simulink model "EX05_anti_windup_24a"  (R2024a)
settings: Solver=VariableStepAuto  StartTime=0.0  StopTime=0.1  MaxStep=1e-5  RelTol=1e-5

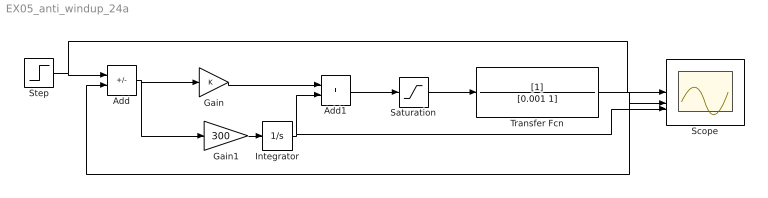
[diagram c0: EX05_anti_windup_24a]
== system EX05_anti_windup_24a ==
  Add : Sum  Inputs=+-
  Add1 : Sum
  Gain : Gain
  Gain1 : Gain  Gain=300
  Integrator : Integrator
  Saturation : Saturate  UpperLimit=60  LowerLimit=-60
  Scope : Scope  NumInputPorts=3
  Step : Step  Time=0.05  Before=100  After=-100  SampleTime=0
  Transfer Fcn : TransferFcn  Denominator=[0.001 1]
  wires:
  Step/1 -> Scope/1, Add/1
  Gain/1 -> Add1/1
  Gain1/1 -> Integrator/1
  Integrator/1 -> Scope/3, Add1/2
  Add1/1 -> Saturation/1
  Saturation/1 -> Transfer Fcn/1
  Transfer Fcn/1 -> Add/2, Scope/2
  Add/1 -> Gain1/1, Gain/1
